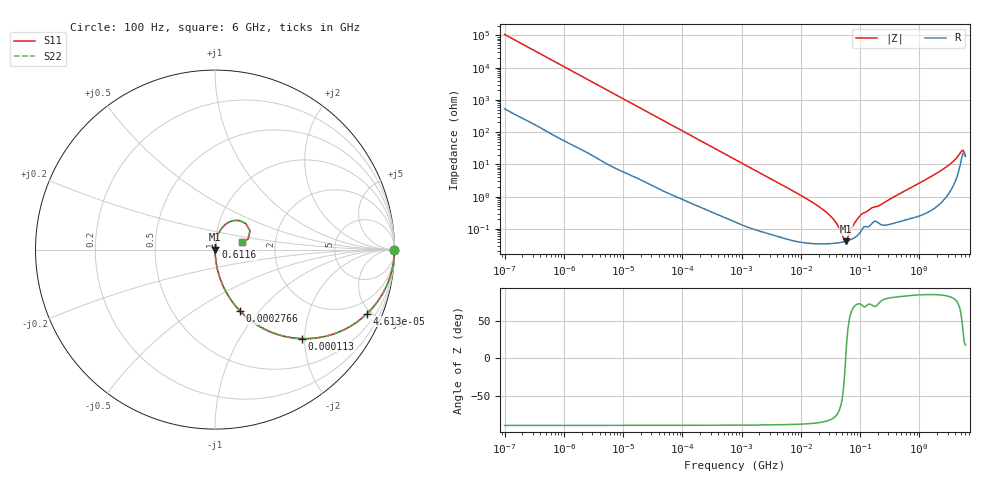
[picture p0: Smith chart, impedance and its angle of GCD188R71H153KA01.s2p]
!Murata Part Number: GCD188R71H153KA01
!These Parameters are Measured in Series Mode Connection
!Data Generated on Jan 08, 2026
!  o--ll--o
!Port1  Port2
!  o------o
!Operation Temp=25[degC], DC Bias Voltage=0[V]
!Freq. Start=100[Hz] Stop=6[GHz] 401[Steps]
# Hz S RI R 50
!Freq.(Hz) S11(Real) S11(Imag) S21(Real) S21(Imag) S12(Real) S12(Imag) S22(Real) S22(Imag)
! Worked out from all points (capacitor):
!   401 points, 100 Hz to 6 GHz, reference 50 ohm
!   read as one part in series: C = 14.8 nF near 109 Hz
!   lowest |Z| = 41.2 mohm at 56.99 MHz (marker M1)
!   series resonance near 57.18 MHz, so ESL is about 520 pH
!   S11 on the Smith chart (normalised r, x): 100 Hz: open; 46.13 kHz: 1.03, -4.74; 113 kHz: 1.01, -1.94; 276.6 kHz: 1.01, -0.80; 611.6 MHz: 1.00, +0.03; 6 GHz: 1.35, +0.11
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100  1 -0.000934  5.5e-06 0.000934  5.5e-06 0.000934  1 -0.000934
2008  0.9996 -0.0186  0.000444 0.0186  0.000444 0.0186  0.9996 -0.0186
11514  0.9883 -0.1047  0.0117 0.1047  0.0117 0.1047  0.9883 -0.1047
40335  0.8784 -0.3237  0.1216 0.3237  0.1216 0.3237  0.8784 -0.3237
46134  0.847 -0.3567  0.153 0.3567  0.153 0.3567  0.847 -0.3567
112960  0.4852 -0.496  0.5148 0.496  0.5148 0.496  0.4852 -0.496
276587  0.1391 -0.3415  0.8609 0.3415  0.8609 0.3415  0.1391 -0.3415
774597  0.0216 -0.1397  0.9784 0.1397  0.9784 0.1397  0.0216 -0.1397
1.555665e7  0.000395 -0.00672  0.9996 0.00672  0.9996 0.00672  0.000395 -0.00672
3.330331e7  0.000356 -0.00225  0.9996 0.00225  0.9996 0.00225  0.000356 -0.00225
3.983537e7  0.000365 -0.00146  0.9996 0.00146  0.9996 0.00146  0.000365 -0.00146
5.211241e7  0.000395 -0.000369  0.9996 0.000369  0.9996 0.000369  0.000395 -0.000369
5.699437e7  0.000411 -1.27e-05  0.9996 1.27e-05  0.9996 1.27e-05  0.000411 -1.27e-05
6.233367e7  0.000432 0.000345  0.9996 -0.000345  0.9996 -0.000345  0.000432 0.000345
8.154455e7  0.000541 0.00147  0.9995 -0.00147  0.9995 -0.00147  0.000541 0.00147
1.066761e8  0.000928 0.00271  0.9991 -0.00271  0.9991 -0.00271  0.000928 0.00271
3.124326e8  0.00144 0.00809  0.9986 -0.00809  0.9986 -0.00809  0.00144 0.00809
6.11557e8  0.00217 0.0159  0.9978 -0.0159  0.9978 -0.0159  0.00217 0.0159
2.562649e9  0.0127 0.0708  0.9873 -0.0708  0.9873 -0.0708  0.0127 0.0708
4.009986e9  0.0448 0.1277  0.9552 -0.1277  0.9552 -0.1277  0.0448 0.1277
5.016141e9  0.1354 0.1622  0.8646 -0.1622  0.8646 -0.1622  0.1354 0.1622
6e9  0.1517 0.04  0.8483 -0.04  0.8483 -0.04  0.1517 0.04
